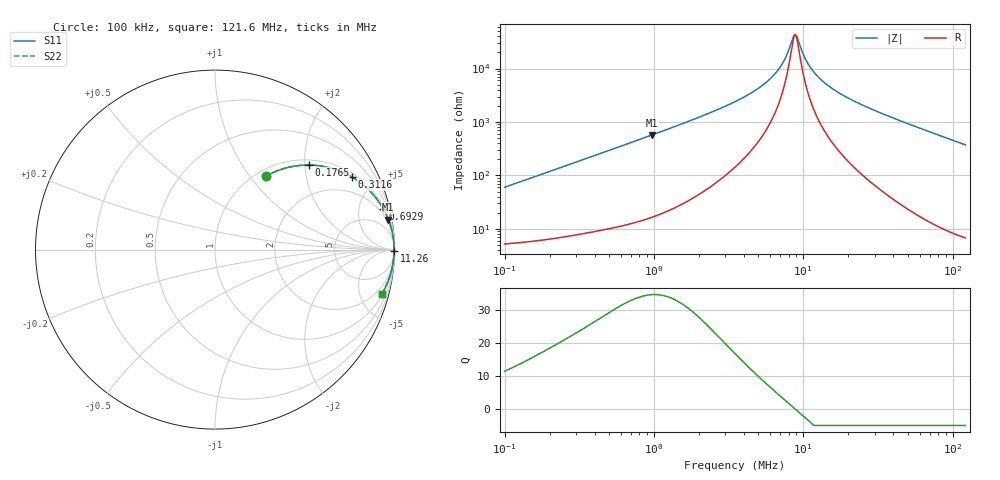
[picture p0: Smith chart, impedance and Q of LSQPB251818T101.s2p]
! LSQPB251818T101  S-PARAMETER MODEL  ( General Type )
! Model Generated by TAIYO YUDEN Corporation (http://www.ty-top.com)
! Version 2.0
! TAIYO YUDEN Control No. 100810NG19SB-FKC
! Copyright(c) 2009 TAIYO YUDEN CO.,LTD. All Rights Reserved.
! Product Description (link to TY-COMPAS)
! https://ds.yuden.co.jp/TYCOMPAS/or/detail?pn=LSQPB251818T101K&u=M
! Products Name : Inductors
! Characteristics :
!  Inductance : 100 uH , SRF(min) : 4.5 MHz , DC Resistance(max) : 4.68 Ohm
!  Rated Current : Saturation :300 mA , Temp Rise : 190 mA (40 degC)
!  Case Size : 2.5 x 1.8 / 0.098 x 0.071 [mm/inch] , Thickness : 1.8 / 0.071 [mm/inch]
!  (Conditions: Temperature = 25 degC , DC Bias Current/Voltage = 0A / 0V)
! External Node Assignments :
!  1  o---GGG---o  2
! GND o---------o GND
! Frequency Range : 0.1MHz  -  121.638923MHz  [ 402 STEP ]
# MHz S RI R 50
! Freq[MHz].  S11 Real  S11 Imag  S21 Real  S21 Imag  S12 Real  S12 Imag  S22 Real  S22 Imag
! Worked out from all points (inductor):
!   401 points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, 100 kHz to 121.6 MHz, reference 50 ohm
!   read as one part in series: L = 94.9 uH near 103.6 kHz
!   highest Q = 34.7 at 971 kHz (marker M1), where L = 93.9 uH
!   self-resonance near 8.782 MHz
!   S11 on the Smith chart (normalised r, x): 100 kHz: 1.10, +1.20; 176.5 kHz: 1.12, +2.10; 311.6 kHz: 1.16, +3.68; 692.9 kHz: 1.25, +8.15; 11.26 MHz: open; 121.6 MHz: 1.14, -7.47
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0.1  0.2819 0.4083  0.7181 -0.4083  0.7181 -0.4083  0.2819 0.4083
0.176525  0.5233 0.471  0.4767 -0.471  0.4767 -0.471  0.5233 0.471
0.31161  0.7627 0.4047  0.2373 -0.4047  0.2373 -0.4047  0.7627 0.4047
0.328662  0.7806 0.3936  0.2194 -0.3936  0.2194 -0.3936  0.7806 0.3936
0.692919  0.937 0.2281  0.063 -0.2281  0.063 -0.2281  0.937 0.2281
0.971009  0.9659 0.1676  0.0341 -0.1676  0.0341 -0.1676  0.9659 0.1676
1.080188  0.972 0.1513  0.028 -0.1513  0.028 -0.1513  0.972 0.1513
3.550168  0.9959 0.0403  0.00409 -0.0403  0.00409 -0.0403  0.9959 0.0403
4.974964  0.9971 0.0234  0.00291 -0.0234  0.00291 -0.0234  0.9971 0.0234
6.379218  0.9975 0.0128  0.00248 -0.0128  0.00248 -0.0128  0.9975 0.0128
7.353073  0.9976 0.00708  0.00235 -0.00708  0.00235 -0.00708  0.9976 0.00708
8.475598  0.9977 0.00153  0.00229 -0.00153  0.00229 -0.00153  0.9977 0.00153
8.782046  0.9977 0.000148  0.00229 -0.000148  0.00229 -0.000148  0.9977 0.000148
9.099574  0.9977 -0.00123  0.00229 0.00123  0.00229 0.00123  0.9977 -0.00123
10.12272  0.9977 -0.00538  0.00231 0.00538  0.00231 0.00538  0.9977 -0.00538
11.2609  0.9976 -0.0096  0.00238 0.0096  0.00238 0.0096  0.9976 -0.0096
11.46267  0.9976 -0.0103  0.00239 0.0103  0.00239 0.0103  0.9976 -0.0103
13.69029  0.9974 -0.0176  0.0026 0.0176  0.0026 0.0176  0.9974 -0.0176
17.24557  0.9969 -0.028  0.00309 0.028  0.00309 0.028  0.9969 -0.028
23.74138  0.9956 -0.045  0.00437 0.045  0.00437 0.045  0.9956 -0.045
37.67347  0.9914 -0.0779  0.00861 0.0779  0.00861 0.0779  0.9914 -0.0779
121.6389  0.9293 -0.2474  0.0707 0.2474  0.0707 0.2474  0.9293 -0.2474
